FUNCTION_BLOCK FB_SignalHandlingIntern IMPLEMENTS ISignalHandling
VAR_INPUT
	bInput		: BOOL;			// Input signal, e.g. sensor signal, enable for fuse
	bEnable		: BOOL;
END_VAR
VAR_OUTPUT
	bOut		: BOOL;
END_VAR

// =========================================================
;
// =========================================================

METHOD PUBLIC M_SetOutput
VAR_INPUT
END_VAR
// =========================================================
	// Out
	
bOut := bInput AND bEnable;

// =========================================================
END_METHOD

END_FUNCTION_BLOCK
